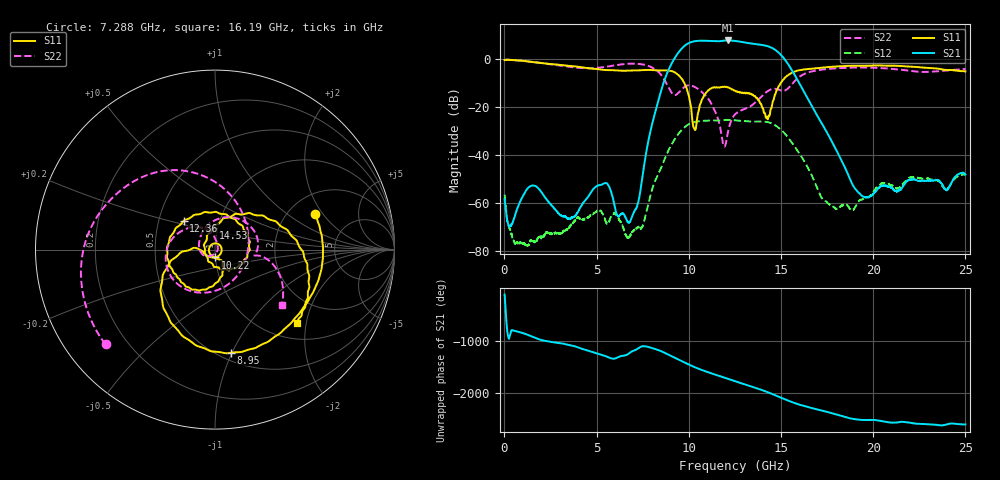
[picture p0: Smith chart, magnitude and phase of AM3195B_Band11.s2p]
!Agilent Technologies,E8364B,MY43040894,A.07.50.67
!Agilent E8364B: A.07.50.67
!Date: Wednesday, July 07, 2021 13:13:52
!Correction: S11(Full 2 Port(1,2))
!S21(Full 2 Port(1,2))
!S12(Full 2 Port(1,2))
!S22(Full 2 Port(1,2))
!S2P File: Measurements: S11, S21, S12, S22:
# Hz S  dB  R 50
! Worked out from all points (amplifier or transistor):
!   8001 points, 10 MHz to 25 GHz, reference 50 ohm
!   highest |S21| = 7.9 dB at 12.11 GHz (marker M1)
!   |S21| within 3 dB of that: 9.663 GHz to 14.48 GHz (4.816 GHz wide, 39.9 % of centre)
!   unconditionally stable (mu >= 1): start of sweep to end of sweep
!   at 4.174 GHz: K = 365401.40, MAG = -56.0 dB, |S12| = -66.6 dB
!   at 12.51 GHz: K = 3.68, MAG = 8.0 dB, |S12| = -25.5 dB
!   at 25 GHz: K = 13701.55, MAG = -44.2 dB, |S12| = -48.4 dB
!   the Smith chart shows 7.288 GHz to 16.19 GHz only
!   S11 on the Smith chart (normalised r, x): 7.288 GHz: 2.75, +1.70; 8.95 GHz: 0.57, -0.99; 10.22 GHz: 1.00, -0.09; 12.36 GHz: 0.67, +0.23; 14.53 GHz: 0.95, +0.23; 16.19 GHz: 1.36, -1.78
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1e7  -0.25 -3.0  -58.35 -127.7  -56.51 147.6  -0.09 -3.8
2.452772e9  -1.88 -149.0  -60.14 60.8  -72.65 -60.6  -1.98 -154.0
4.177082e9  -3.25 144.9  -61.13 -70.8  -66.61 25.8  -3.61 98.5
5.626502e9  -4.45 93.9  -52.44 126.2  -68.32 -43.7  -2.92 -15.9
7.288338e9  -4.54 19.8  -58.63 -55.9  -70.29 -152.2  -1.86 -139.1
8.341041e9  -4.60 -38.2  -17.39 -98.0  -48.09 162.7  -5.13 130.4
8.950172e9  -4.71 -81.1  -3.50 165.2  -37.23 56.8  -12.40 46.8
9.596789e9  -7.91 -137.2  4.41 55.3  -29.62 -51.2  -12.64 -92.6
1.022154e10  -27.20 -90.7  7.48 -47.0  -26.37 -148.7  -11.18 -173.0
1.063075e10  -18.46 -65.6  7.83 -105.4  -25.78 155.8  -13.13 154.2
1.116179e10  -12.23 -111.0  7.78 -172.0  -25.52 91.8  -17.68 116.8
1.210828e10  -11.72 170.4  7.95 80.7  -25.27 -12.1  -30.90 -106.5
1.236443e10  -12.51 137.7  7.88 50.7  -25.39 -40.7  -24.53 -142.3
1.2505e10  -13.06 118.8  7.76 34.3  -25.47 -56.1  -22.97 -154.0
1.354208e10  -15.32 -22.6  6.48 -83.4  -26.01 -169.2  -18.41 126.3
1.410436e10  -22.37 -116.7  5.88 -152.1  -26.03 122.8  -14.29 69.7
1.452607e10  -18.32 95.6  4.78 149.5  -26.86 66.4  -12.35 25.4
1.523516e10  -7.50 13.8  -0.30 45.8  -31.25 -27.0  -12.90 -8.2
1.619415e10  -4.24 -41.6  -12.72 -70.8  -41.70 -127.8  -6.32 -39.5
1.667208e10  -3.85 -58.6  -19.45 -115.9  -48.53 -172.1  -5.00 -62.2
2.083604e10  -2.64 -153.5  -53.19 -24.6  -52.04 -21.6  -3.80 156.0
2.5e10  -5.01 97.1  -48.12 -65.9  -48.40 -68.4  -3.96 -28.8
